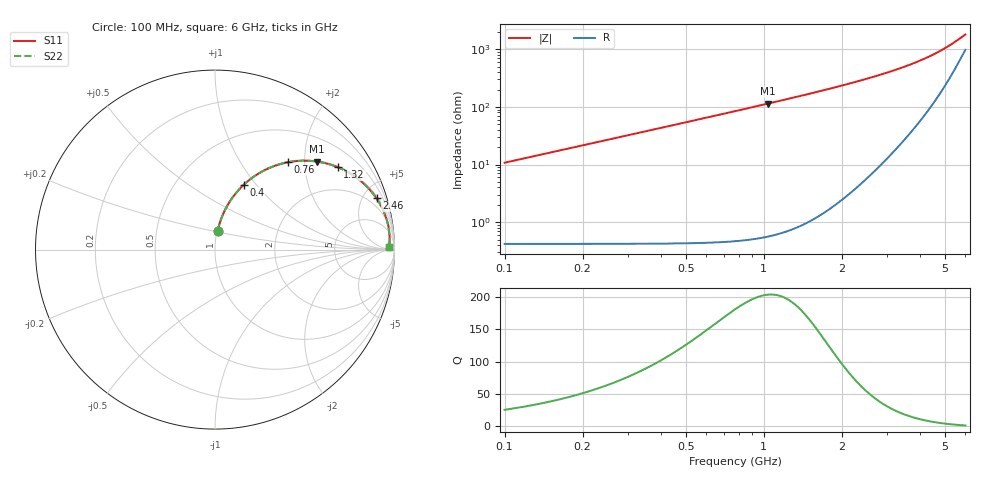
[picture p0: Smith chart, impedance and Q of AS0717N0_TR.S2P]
!AVX Corporation
! AVX AS0717N0*TR
! DESCRIPTION: SQUARE AIR CORE INDUCTOR, 17nH, 6 turns
# MHZ S MA R 50
!Freq  MagS11  AngS11  MagS21  AngS21  MagS12  AngS12  MagS22  AngS22
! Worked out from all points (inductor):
!   296 points, 100 MHz to 6 GHz, reference 50 ohm
!   read as one part in series: L = 17.1 nH near 120 MHz
!   highest Q = 203 at 1.04 GHz (marker M1), where L = 17.5 nH
!   S11 on the Smith chart (normalised r, x): 100 MHz: 1.01, +0.21; 400 MHz: 1.01, +0.86; 760 MHz: 1.02, +1.65; 1.32 GHz: 1.03, +2.96; 2.46 GHz: 1.19, +6.24; 6 GHz: 52, +26
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100  0.1061 81.6  0.9902 -6.1  0.9902 -6.1  0.1061 81.6
120  0.127 80.8  0.9878 -7.3  0.9878 -7.3  0.127 80.8
160  0.1683 78.9  0.9816 -9.7  0.9816 -9.7  0.1683 78.9
220  0.2287 75.7  0.9694 -13.3  0.9694 -13.3  0.2287 75.7
260  0.2676 73.5  0.9595 -15.6  0.9595 -15.6  0.2676 73.5
300  0.3052 71.4  0.9483 -17.9  0.9483 -17.9  0.3053 71.4
400  0.3935 66.2  0.9155 -23.3  0.9155 -23.3  0.3935 66.2
480  0.4574 62.2  0.8855 -27.3  0.8855 -27.3  0.4574 62.2
560  0.5152 58.4  0.8534 -31.2  0.8534 -31.2  0.5152 58.4
660  0.579 54.1  0.8117 -35.6  0.8117 -35.6  0.579 54.1
760  0.6341 50.1  0.7697 -39.6  0.7697 -39.6  0.6341 50.1
900  0.6983 45.2  0.7123 -44.5  0.7123 -44.5  0.6983 45.2
1040  0.7498 40.9  0.658 -48.9  0.658 -48.9  0.7498 40.9
1100  0.7686 39.2  0.636 -50.5  0.636 -50.5  0.7686 39.2
1320  0.8242 33.8  0.5619 -55.9  0.5619 -55.9  0.8242 33.8
1660  0.8809 27.4  0.4671 -62.2  0.4671 -62.2  0.8809 27.4
2080  0.922 21.6  0.3768 -67.8  0.3768 -67.8  0.922 21.6
2460  0.944 17.6  0.3136 -71.4  0.3136 -71.4  0.944 17.6
3060  0.9631 12.9  0.2376 -75.1  0.2376 -75.1  0.9632 12.9
4040  0.9746 7.6  0.1515 -77.2  0.1515 -77.2  0.9746 7.6
5020  0.9749 3.8  0.09286 -73.1  0.09286 -73.1  0.9749 3.8
6000  0.9698 0.9  0.05377 -56.2  0.05377 -56.2  0.9698 0.9
